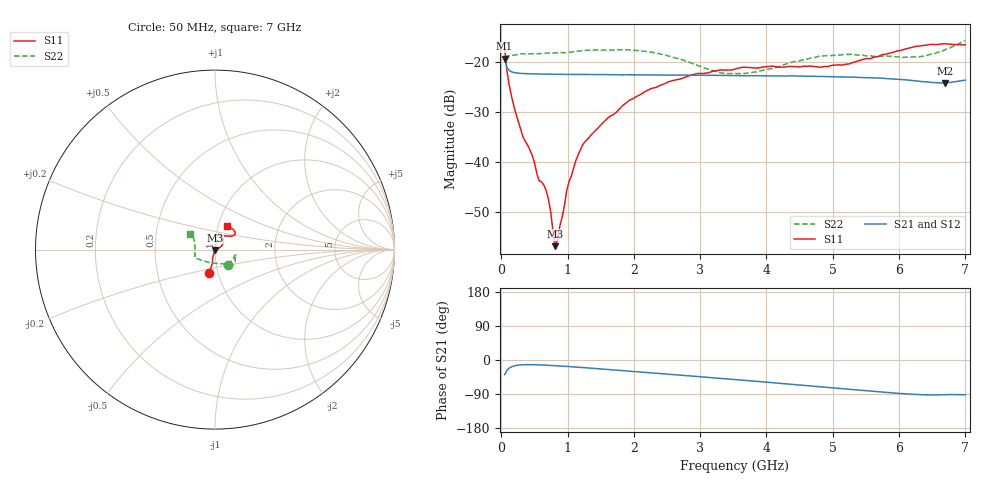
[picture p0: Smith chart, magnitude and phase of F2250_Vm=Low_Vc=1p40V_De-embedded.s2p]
! Integrated Device Technology
! Corporate Headquarters
! 6024 Silver Creek Valley Road
! San Jose, CA 95138  USA
! Phone:  1-408-284-8200
! Toll Free:  1-800-223-1366
! Webpage:  http://www.idt.com/
! Timing and RF Division
! 515 Groton Road, Suite 102
! Westford, MA 01886-6024
! Device:  F2250
! Description: Voltage Variable RF Attenuator
! Frequency:  50.0 -  6000.00 MHz
! Package:  3x3 mm Thin QFN Plastic Package: 16 pin
! Ports:  2 RF, 3 DC
!  Pin  1  = GND
!  Pin  2  = NC
!  Pin  3  = RF1  = Port 1
!  Pin  4  = NC
!  Pin  5  = GND
!  Pin  6  = GND
!  Pin  7  = GND
!  Pin  8  = GND
!  Pin  9  = NC
!  Pin 10  = RF2  = Port 2
!  Pin 11  = NC
!  Pin 12  = GND
!  Pin 13  = GND
!  Pin 14  = VCNTRL
!  Pin 15  = VDD
!  Pin 16  = VMODE
! Vcntrl:  1.400 Volts
! Vmode:  +0.000 Volts
! Vdd:  +3.30  Volts
! Current:  1.192 mA
! Data:  The device was measured on a the F2250 evaluation board which has
!  individual transmission lines to the RF pins.  Data was collected
!  using a calibrated network analyzer.  The evaluation board was
!  de-embedded using a TRL calibration technique.
!  The reference plane is the edge of the package pin.
! Misc:  SN 10
!  Action Tracker AT0258
! Date Measured:  2014-11-26
! Date:  2015-10-15  MJV
! Note:
!  Integrated Device Technology supplies this data as a sample of measured
!  data at the package pin for this product.  Your particular data for this
!  product may vary.
!  Data was taken at 25 degrees C.
!  Integrated Device Technology reserves the right to change this data at anytime.
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# GHz S dB R 50
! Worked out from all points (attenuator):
!   201 points, 50 MHz to 7 GHz, reference 50 ohm
!   highest |S21| = -19.36 dB at 50 MHz (marker M1); lowest = -24.2 dB at 6.687 GHz (marker M2)
!   lowest |S11| = -56.8 dB at 814.5 MHz (marker M3), VSWR 1.00, Z = 50 - j0.141 ohm
!   |S11| at or under -10 dB: start of sweep to end of sweep
!   |S22| runs from -22.4 to -15.7 dB; largest |S21 - S12| = 0.00027
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0.05  -17.41 -104.3  -19.36 -38.9  -19.34 -38.8  -19.13 -50.1
0.1195  -24.64 -102.9  -21.70 -21.3  -21.71 -21.3  -18.81 -19.1
0.189  -28.80 -106.1  -22.12 -15.7  -22.11 -15.7  -18.66 -14.5
0.328  -35.03 -108.7  -22.33 -12.5  -22.33 -12.5  -18.37 -13.2
0.467  -38.68 -114.8  -22.40 -12.3  -22.40 -12.3  -18.40 -14.3
0.57125  -43.72 -113.6  -22.43 -12.9  -22.44 -12.9  -18.37 -16.6
0.6755  -45.68 -101.1  -22.45 -13.7  -22.45 -13.7  -18.27 -18.6
0.745  -49.97 -95.8  -22.46 -14.4  -22.46 -14.4  -18.25 -20.2
0.8145  -56.80 -77.6  -22.48 -15.1  -22.50 -15.1  -18.20 -21.8
0.84925  -55.42 -47.9  -22.50 -15.4  -22.49 -15.4  -18.17 -22.7
1.023  -43.86 -12.2  -22.50 -17.3  -22.49 -17.3  -18.09 -25.6
1.2315  -36.48 9.1  -22.51 -19.9  -22.52 -19.9  -17.74 -29.7
1.857  -28.44 27.0  -22.59 -28.2  -22.58 -28.2  -17.57 -37.5
2.37825  -24.80 38.3  -22.63 -35.4  -22.62 -35.4  -18.34 -44.1
2.93425  -22.40 53.7  -22.68 -43.2  -22.69 -43.2  -20.57 -58.7
3.525  -21.43 68.3  -22.74 -51.7  -22.73 -51.7  -22.34 -96.3
4.7065  -20.93 70.2  -22.90 -69.0  -22.88 -69.1  -19.18 -152.0
5.22775  -20.45 53.8  -23.02 -77.0  -23.03 -76.9  -18.51 -160.3
5.85325  -18.27 38.2  -23.38 -86.1  -23.38 -86.1  -18.89 -171.6
6.33975  -16.77 39.4  -23.93 -91.5  -23.93 -91.6  -18.92 169.8
6.68725  -16.37 47.6  -24.20 -91.6  -24.21 -91.5  -17.59 153.0
7  -16.60 62.7  -23.66 -91.8  -23.68 -91.8  -15.73 147.9
